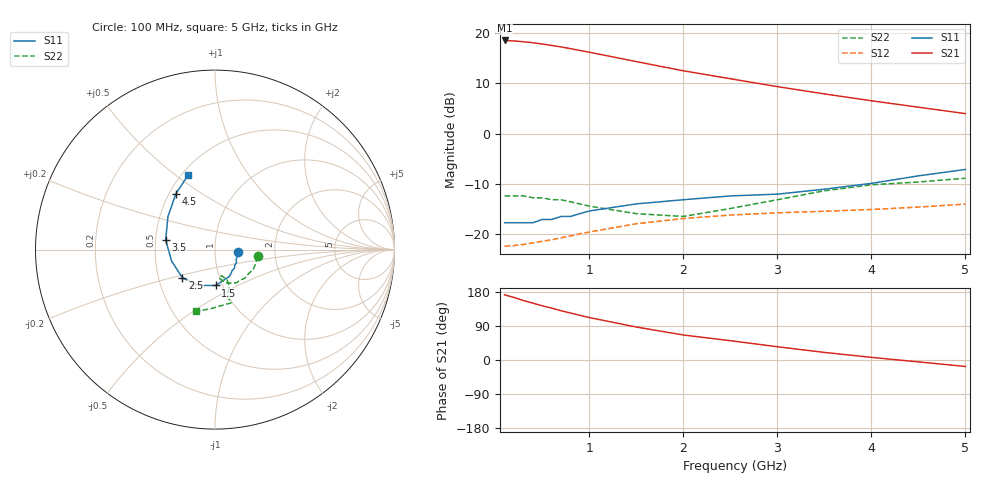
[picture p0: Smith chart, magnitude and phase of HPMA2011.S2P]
! HPMA-2011
! Typical S-Parameters, Z  = 50 , T  = 25 C, I  = 25mA
# ghz s ma r 50
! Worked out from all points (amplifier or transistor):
!   18 points, 100 MHz to 5 GHz, reference 50 ohm
!   highest |S21| = 18.5 dB at 100 MHz (marker M1)
!   |S21| within 3 dB of that: start of sweep to 1.178 GHz
!   unconditionally stable (mu >= 1): start of sweep to end of sweep
!   at 400 MHz: K = 1.06, MAG = 18.4 dB, |S12| = -21.7 dB
!   at 1 GHz: K = 1.03, MAG = 16.8 dB, |S12| = -19.6 dB
!   at 5 GHz: K = 1.12, MAG = 6.9 dB, |S12| = -14.0 dB
!   S11 on the Smith chart (normalised r, x): 100 MHz: 1.30, -0.04; 1.5 GHz: 0.93, -0.39; 2.5 GHz: 0.66, -0.22; 3.5 GHz: 0.57, +0.07; 4.5 GHz: 0.54, +0.39; 5 GHz: 0.54, +0.55
0.1  0.13 -6.0  8.43 172.0  0.076 4.0  0.24 -9.0
0.2  0.13 -12.0  8.33 165.0  0.077 8.0  0.24 -18.0
0.3  0.13 -19.0  8.19 157.0  0.079 11.0  0.24 -27.0
0.4  0.13 -25.0  8 150.0  0.082 14.0  0.23 -36.0
0.5  0.14 -31.0  7.77 143.0  0.085 17.0  0.23 -44.0
0.6  0.14 -38.0  7.52 137.0  0.088 19.0  0.22 -51.0
0.7  0.15 -44.0  7.27 130.0  0.092 21.0  0.22 -57.0
0.8  0.15 -50.0  6.99 124.0  0.096 22.0  0.21 -63.0
0.9  0.16 -56.0  6.71 118.0  0.101 23.0  0.2 -69.0
1  0.17 -62.0  6.44 112.0  0.105 24.0  0.19 -73.0
1.5  0.2 -89.0  5.2 87.0  0.127 25.0  0.16 -82.0
2  0.22 -115.0  4.21 66.0  0.143 23.0  0.15 -76.0
2.5  0.24 -139.0  3.51 51.0  0.155 23.0  0.18 -68.0
3  0.25 -165.0  2.93 35.0  0.163 20.0  0.22 -69.0
3.5  0.28 169.0  2.48 20.0  0.169 19.0  0.27 -75.0
4  0.32 145.0  2.12 7.0  0.176 19.0  0.31 -73.0
4.5  0.38 125.0  1.83 -5.0  0.186 19.0  0.33 -94.0
5  0.44 110.0  1.58 -17.0  0.199 19.0  0.36 -107.0
